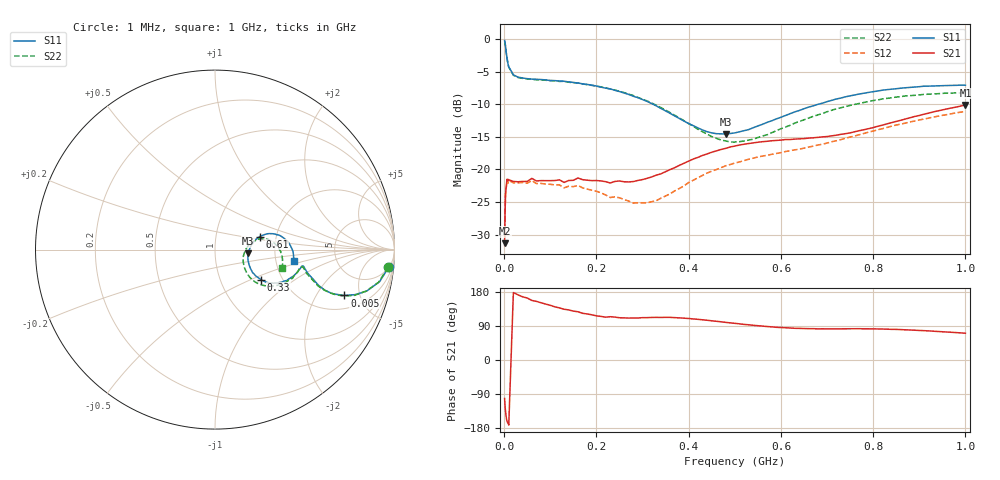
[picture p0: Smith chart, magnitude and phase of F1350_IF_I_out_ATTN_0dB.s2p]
! S-parameters for IF_I+ & IF_I- IDT F1350 DPD Demodulator
! Date Measured:  2015-11-25  RGG
!  Port 1 = Pin 19 = IF_I+
!  Port 2 = Pin 20 = IF_I-
! State: 0 dB attenuation (Gain = Gmax - 0 dB)
! IF Frequency:  1 MHz to 1000 MHz
! RF_INX, RF_INY, IF_Q+, and IF_Q- terminated
! 2300 MHz, 0 dBm signal applied to LO_IN
! Vcc = +5.00 Volts  Icc = approx 275 mA.
! NOTES:  The device was measured on a custom printed circuit evaluation board with individual 50 ohm
!  microstrip lines to the RF and LO pins. The IF outputs are normally connected to balun
!  transformers, which convert the balanced IF output signals to single ended (SE) 50 ohm signals
!  for normal test purposes. For these measurements, to measure the IFI+ and IFI- output SE s-parameters,
!  the chokes associated with the IFI+ and IFI- outputs were removed and a pair of pigtailed
!  50 ohm coaxial lines were soldered to the PCB at these points. 5.00 volt bias was provided
!  to these pins via external bias tees. Data was collected using a calibrated vector
!  network analyzer.  The pigtailed 50 ohm coaxial lines were de-embedded using reference
!  plane extensions. 100 ohm microstrip lines of length 386 mils and 218 mils for the IF_I+ and IF_I-
!  signals, respectively, were de-embedded using Agilent ADS, yielding the reference plane at the IC edge.
!  Only IFI+ and IFI- outputs were measured. IF_Q+ and IF_Q- should be identical.
!  This data is single-ended relative to ports IF_I+ and IF_I- (reference impedance = 50 ohms)
!  Common mode or differential S-parameters may be extracted from this data with a linear simulator.
# mhz S db R 50
! freq  dbS11  angS11  dbS21  angS21  dbS12  angS12  dbS22  angS22
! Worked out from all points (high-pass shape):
!   109 points, 1 MHz to 1 GHz, reference 50 ohm
!   highest |S21| = -10.12 dB at 1 GHz (marker M1); lowest = -31.3 dB at 1 MHz (marker M2)
!   |S21| within 3 dB of the highest: 824.3 MHz to end of sweep
!   lowest |S11| = -14.6 dB at 480 MHz (marker M3), VSWR 1.46, Z = 72.8 - j3.12 ohm
!   |S11| at or under -10 dB: 322.6 MHz to 680.9 MHz (358.3 MHz wide, 71.4 % of centre)
!   |S22| runs from -15.8 to -0.3 dB; largest |S21 - S12| = 0.066
!   S11 on the Smith chart (normalised r, x): 1 MHz: 5, -19; 5 MHz: 2.90, -3.57; 330 MHz: 1.56, -0.58; 610 MHz: 1.64, +0.26; 1 GHz: 2.51, -0.40
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1  -0.23 -5.6  -31.32 -101.7  -31.75 -106.2  -0.27 -5.8
2  -0.59 -11.0  -26.53 -122.6  -26.67 -120.9  -0.64 -11.3
3  -1.15 -15.3  -23.78 -135.4  -23.87 -134.5  -1.17 -15.3
5  -2.33 -19.5  -22.29 -155.1  -22.55 -151.0  -2.34 -19.8
6  -2.87 -20.3  -21.52 -160.7  -21.79 -159.5  -2.87 -20.5
8  -3.70 -20.3  -21.49 -166.7  -22.13 -166.4  -3.72 -20.4
10  -4.27 -19.1  -21.57 -171.8  -21.68 -171.7  -4.30 -19.4
20  -5.50 -14.1  -21.84 178.0  -22.04 178.7  -5.56 -14.5
50  -6.08 -10.6  -21.83 163.6  -22.10 165.2  -6.12 -11.0
60  -6.15 -10.8  -21.37 157.2  -21.70 158.7  -6.18 -11.4
130  -6.49 -15.9  -21.99 134.0  -22.81 136.1  -6.48 -16.7
170  -6.87 -19.8  -21.56 123.2  -22.81 125.0  -6.88 -21.1
280  -8.78 -30.7  -21.85 110.9  -25.15 114.3  -8.66 -33.7
330  -10.26 -33.1  -20.86 112.5  -24.78 123.6  -10.17 -38.1
340  -10.65 -33.1  -20.67 112.3  -24.38 124.9  -10.51 -38.6
430  -13.94 -21.5  -17.85 106.1  -20.91 125.0  -14.20 -32.0
480  -14.56 -6.3  -16.77 99.3  -19.44 119.7  -15.62 -18.2
510  -14.23 2.1  -16.26 95.5  -18.85 116.0  -15.74 -8.7
610  -11.72 16.3  -15.41 85.1  -17.25 106.8  -13.50 11.2
670  -10.25 16.7  -15.14 82.7  -16.43 103.5  -11.86 13.4
840  -7.69 5.3  -12.82 80.9  -13.36 93.5  -9.01 1.3
1000  -7.09 -8.4  -10.12 70.7  -11.09 78.3  -8.21 -15.3
